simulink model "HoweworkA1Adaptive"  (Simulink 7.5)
settings: Solver=ode45  StartTime=0.0  StopTime=10.0  RelTol=1e-3

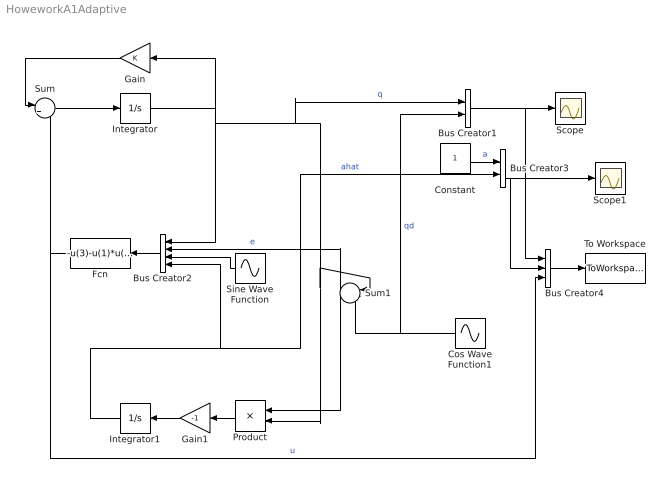
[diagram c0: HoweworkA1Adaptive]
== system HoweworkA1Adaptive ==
  Bus Creator1 : BusCreator  Inputs=2
  Bus Creator2 : BusCreator
  Bus Creator3 : BusCreator  Inputs=2
  Bus Creator4 : BusCreator  Inputs=3
  Constant : Constant  OutDataType=fixdt(1, 16)  OutScaling=2^0
  Cos Wave Function1 : Sin  Amplitude=1  Bias=0  Frequency=1  Phase=pi/2  Samples=10  SampleTime=0
  Fcn : Fcn  Expr=-u(3)-u(1)*u(4)+10*(u(2))
  Gain : Gain  ParameterDataType=fixdt(1, 16)  ParameterScaling=2^0  OutDataType=fixdt(1, 16)  OutScaling=2^0
  Gain1 : Gain  Gain=-1  ParameterDataType=fixdt(1, 16)  ParameterScaling=2^0  OutDataType=fixdt(1, 16)  OutScaling=2^0
  Integrator : Integrator
  Integrator1 : Integrator
  Product : Product  OutDataType=fixdt(1, 16)  OutScaling=2^0
  Scope : Scope
  Scope1 : Scope
  Sine Wave Function : Sin  Amplitude=1  Bias=0  Frequency=1  Phase=0  Samples=10  SampleTime=0
  Sum : Sum  Inputs=|++  OutDataType=fixdt(1, 16)  OutScaling=2^0
  Sum1 : Sum  Inputs=|-+  OutDataType=fixdt(1, 16)  OutScaling=2^0
  To Workspace : ToWorkspace  VariableName=ICP  SampleTime=-1  SaveFormat=Structure With Time
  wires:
  Integrator/1 -> Gain/1, Bus Creator2/1, Bus Creator1/1, Sum1/1, Product/2  "q"
  Sum/1 -> Integrator/1
  Gain/1 -> Sum/1
  Bus Creator1/1 -> Scope/1, Bus Creator4/1
  Fcn/1 -> Sum/2, Bus Creator4/3  "u"
  Bus Creator2/1 -> Fcn/1
  Cos Wave Function1/1 -> Sum1/2, Bus Creator1/2  "qd"
  Sum1/1 -> Bus Creator2/2, Product/1  "e"
  Product/1 -> Gain1/1
  Gain1/1 -> Integrator1/1
  Integrator1/1 -> Bus Creator3/2, Bus Creator2/4  "ahat"
  Bus Creator3/1 -> Scope1/1, Bus Creator4/2
  Sine Wave Function/1 -> Bus Creator2/3
  Constant/1 -> Bus Creator3/1  "a"
  Bus Creator4/1 -> To Workspace/1
